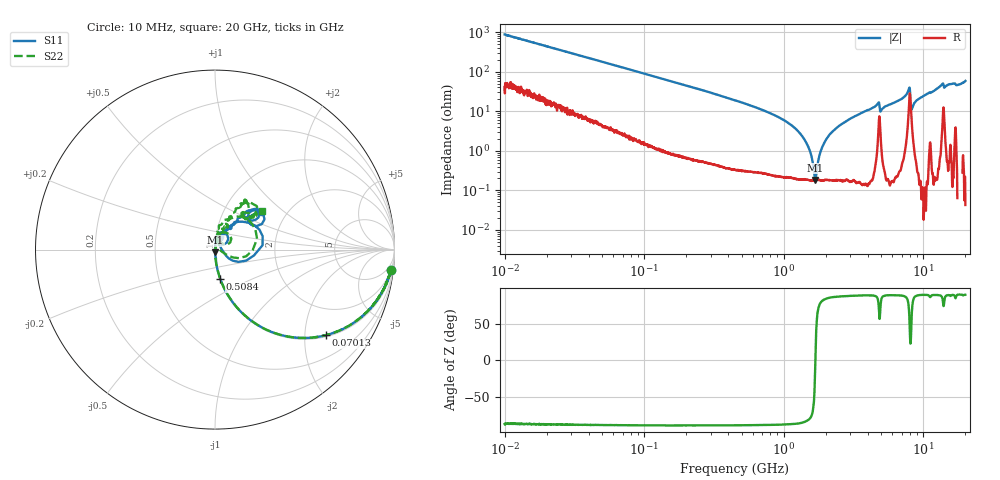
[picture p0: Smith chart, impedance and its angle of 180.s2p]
!Keysight Technologies,P5008B,MY61100088,A.16.20.02
!Date: Friday, August 30, 2024 13:43:54
!Correction: S11(C  2-Port  )
!S21(C  2-Port  )
!S12(C  2-Port  )
!S22(C  2-Port  )
!S2P File: Measurements: S11, S21, S12, S22:Log Frequency Sweep
# Hz S  MA  R 50
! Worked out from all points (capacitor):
!   1601 points, 10 MHz to 20 GHz, reference 50 ohm
!   read as one part in series: C = 18.2 pF near 10.39 MHz
!   lowest |Z| = 183 mohm at 1.683 GHz (marker M1)
!   series resonance near 1.684 GHz, so ESL is about 490 pH
!   S11 on the Smith chart (normalised r, x): 10 MHz: 2, -17; 70.13 MHz: 1.05, -2.55; 508.4 MHz: 1.00, -0.34; 20 GHz: 1.50, +0.70
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1e7  0.9888 -6.5  0.1128 80.8  0.1128 80.9  0.9883 -6.5
3.555162e7  0.9193 -21.6  0.3673 66.7  0.3671 66.7  0.9191 -21.6
7.012759e7  0.7802 -37.7  0.6107 51.2  0.6104 51.2  0.7801 -37.7
1.263918e8  0.5775 -54.0  0.808 35.1  0.8076 35.1  0.5778 -54.0
4.472136e8  0.1903 -78.5  0.9787 10.5  0.9782 10.5  0.1903 -78.6
5.084168e8  0.1658 -79.9  0.9832 9.0  0.9827 9.0  0.1656 -80.0
1.051673e9  0.06224 -84.9  0.9961 2.6  0.9957 2.5  0.06216 -86.0
1.589917e9  0.0199 -84.2  0.9983 -0.4  0.9978 -0.4  0.02015 -86.2
1.683186e9  0.01457 -85.8  0.9984 -0.8  0.9979 -0.8  0.01471 -80.6
1.97824e9  0.002714 1.3  0.9985 -2.0  0.9981 -2.0  0.001358 -17.3
2.134466e9  0.007291 71.0  0.9987 -2.6  0.9982 -2.6  0.006891 70.8
2.313997e9  0.01303 81.1  0.9986 -3.2  0.9982 -3.2  0.01237 73.6
2.838428e9  0.03092 86.6  0.9985 -4.9  0.998 -4.9  0.03046 74.6
4.674208e9  0.098 74.7  0.9855 -11.3  0.985 -11.4  0.09971 69.7
5.067356e9  0.05471 78.1  0.9931 -9.9  0.9925 -9.9  0.05761 67.6
5.652411e9  0.07591 76.7  0.9972 -12.2  0.9968 -12.3  0.07909 74.3
7.770776e9  0.2157 46.1  0.9309 -22.9  0.9306 -23.0  0.2115 58.8
8.545299e9  0.04308 41.3  0.9898 -15.6  0.9897 -15.7  0.04087 63.9
9.264046e9  0.07926 57.4  0.9987 -19.4  0.9984 -19.6  0.07992 75.9
1.335558e10  0.2965 47.9  0.9543 -33.5  0.9537 -33.7  0.2946 59.2
1.801527e10  0.245 46.6  0.9777 -42.6  0.9774 -42.8  0.2398 48.4
2e10  0.3316 38.8  0.9465 -50.7  0.9462 -50.9  0.3388 39.4
